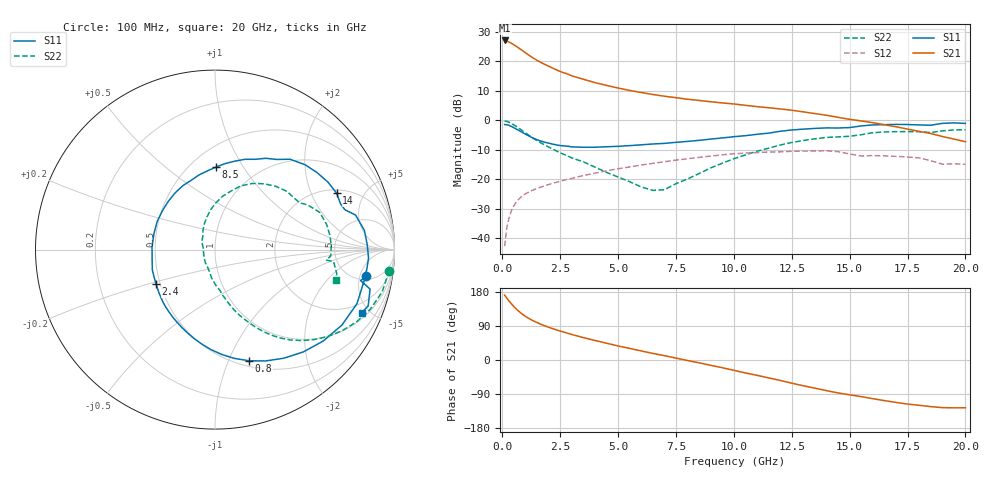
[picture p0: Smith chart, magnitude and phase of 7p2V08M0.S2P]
! Infineon Technologies  Discrete & RF Semiconductors
! bfp620
! VCE =  2.0 V,  IC =  8.0 mA
! Common Emitter S-Parameters:  Sep 2002
# GHz  S  MA  R  50
!  f  S11  S21  S12  S22
! GHz  MAG  ANG  MAG  ANG  MAG  ANG  MAG  ANG
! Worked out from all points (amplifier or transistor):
!   59 points, 100 MHz to 20 GHz, reference 50 ohm
!   highest |S21| = 27.1 dB at 100 MHz (marker M1)
!   |S21| within 3 dB of that: start of sweep to 790 MHz
!   unconditionally stable (mu >= 1): 4.273 GHz to 11.05 GHz; 17.11 GHz to end of sweep
!   at 1 GHz: K = 0.44, MSG = 23.9 dB, |S12| = -24.9 dB
!   at 5.5 GHz: K = 1.05, MAG = 11.6 dB, |S12| = -15.7 dB
!   at 20 GHz: K = 1.33, MAG = 0.4 dB, |S12| = -14.9 dB
!   S11 on the Smith chart (normalised r, x): 100 MHz: 5.67, -6.18; 800 MHz: 0.56, -1.19; 2.4 GHz: 0.47, -0.21; 8.5 GHz: 0.66, +0.77; 14 GHz: 2.18, +3.10; 20 GHz: 1.33, -4.47
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0.1  0.8518 -10.1  22.67 171.3  0.0074 75.7  0.9778 -6.9
0.2  0.8464 -20.9  22.11 162.9  0.0156 76.9  0.9607 -14.2
0.3  0.8225 -30.8  21.24 155.1  0.0231 73.2  0.9278 -20.9
0.4  0.7894 -40.2  20.22 147.9  0.0298 69.2  0.8859 -27.0
0.5  0.7531 -49.2  19.13 141.1  0.0358 65.4  0.8398 -32.6
0.6  0.7166 -57.6  18.05 134.9  0.0411 62.0  0.7923 -37.7
0.8  0.6477 -73.0  15.95 124.0  0.05 56.4  0.6997 -46.4
0.9  0.6157 -79.9  14.97 119.4  0.0537 54.1  0.6562 -50.1
1.1  0.5575 -92.3  13.17 111.3  0.06 50.4  0.5772 -56.1
1.4  0.4885 -108.4  11.01 101.6  0.0679 46.7  0.4811 -62.8
1.6  0.4559 -117.8  9.926 96.1  0.0726 44.9  0.4312 -66.3
1.9  0.4215 -130.6  8.668 88.7  0.0795 42.9  0.372 -70.9
2.4  0.3809 -149.5  7.013 78.3  0.0908 39.9  0.2956 -76.8
3.5  0.3511 177.9  4.984 59.1  0.1164 33.5  0.199 -88.6
5  0.3643 143.6  3.541 37.1  0.1516 23.3  0.1099 -111.0
7  0.4087 108.7  2.573 11.5  0.1997 7.8  0.0669 170.9
8.5  0.46 89.3  2.18 -7.5  0.2367 -5.9  0.126 122.2
10.5  0.5516 65.8  1.805 -34.2  0.2794 -27.9  0.2602 89.0
13.5  0.7329 30.9  1.308 -74.3  0.3035 -60.9  0.4879 46.4
14  0.7471 24.9  1.225 -80.8  0.3059 -67.4  0.5156 39.0
17  0.8568 -3.1  0.782 -112.0  0.2459 -91.9  0.6453 6.8
20  0.8897 -23.3  0.436 -126.1  0.1806 -104.1  0.6964 -14.3
